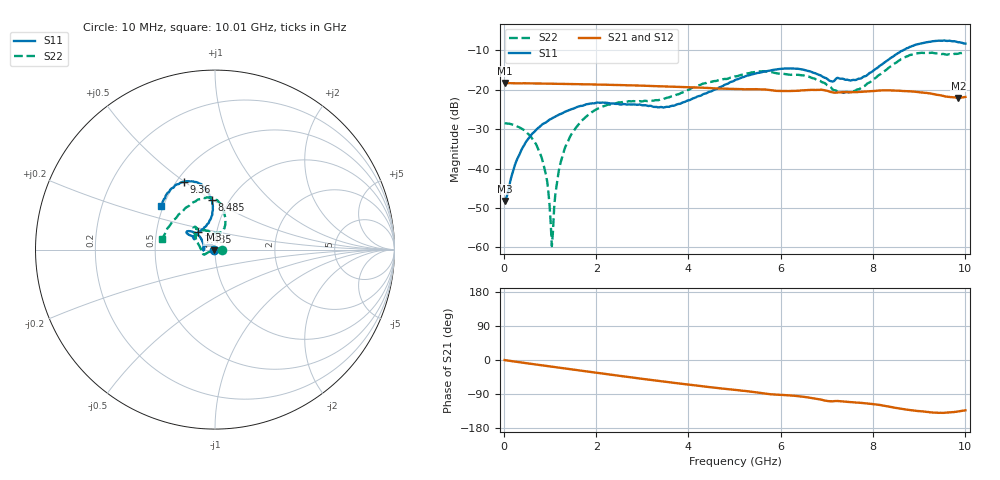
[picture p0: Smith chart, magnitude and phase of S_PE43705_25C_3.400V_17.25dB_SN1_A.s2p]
! Device ID: PE43705
! Serial: 1
! Insertion: A
! Impedance: 50 ohm
! Temp: 25C
! VDD: 3.400V
! Attenuation Step: 17.25dB
#  Hz  S  RI  R  50
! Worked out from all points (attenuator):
!   401 points, 10 MHz to 10.01 GHz, reference 50 ohm
!   highest |S21| = -18.31 dB at 10 MHz (marker M1); lowest = -22.1 dB at 9.86 GHz (marker M2)
!   lowest |S11| = -48.2 dB at 10 MHz (marker M3), VSWR 1.01, Z = 49.6 + j0.0457 ohm
!   |S11| at or under -10 dB: start of sweep to 8.659 GHz
!   |S22| runs from -59.7 to -10.4 dB; largest |S21 - S12| = 0.0015
!   S11 on the Smith chart (normalised r, x): 10 MHz: 0.99, +0.00; 7.435 GHz: 0.82, +0.16; 8.485 GHz: 0.83, +0.49; 9.36 GHz: 0.55, +0.50; 10.01 GHz: 0.49, +0.27
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1e7  -0.00385 0.000461  0.1214 -0.000448  0.1216 -0.000501  0.0375 1.82e-05
3.35e8  -0.00617 0.0139  0.1199 -0.0124  0.1197 -0.0123  0.033 0.00418
7.1e8  -0.0187 0.0255  0.1173 -0.0254  0.1173 -0.0253  0.0184 0.00605
8.85e8  -0.0268 0.0268  0.1155 -0.0314  0.1155 -0.0313  0.00893 0.0036
1.01e9  -0.0324 0.0273  0.1138 -0.0356  0.1139 -0.0355  0.00158 0.00133
1.035e9  -0.0334 0.0272  0.1134 -0.0363  0.1135 -0.0363  0.000146 0.00103
1.085e9  -0.0358 0.0269  0.1128 -0.0377  0.1128 -0.0378  -0.00315 -0.000261
1.16e9  -0.039 0.0266  0.1119 -0.0401  0.1118 -0.0401  -0.00732 -0.00166
1.26e9  -0.0432 0.0254  0.1104 -0.0433  0.1105 -0.0432  -0.0133 -0.00406
1.435e9  -0.0513 0.0227  0.1076 -0.0487  0.1077 -0.0486  -0.0242 -0.00858
1.685e9  -0.0601 0.0168  0.1032 -0.0558  0.1033 -0.0559  -0.0376 -0.0153
2.26e9  -0.0676 0.000283  0.0912 -0.0709  0.0912 -0.0707  -0.0584 -0.0277
3.36e9  -0.0596 0.0035  0.063 -0.0911  0.0628 -0.0909  -0.0739 -0.00399
5.01e9  -0.1001 0.0865  0.0196 -0.1002  0.0197 -0.1001  -0.1136 0.0937
6.01e9  -0.1535 0.1016  -0.00328 -0.0962  -0.00292 -0.0961  -0.104 0.1206
6.685e9  -0.1445 0.0819  -0.0182 -0.0978  -0.0184 -0.0977  -0.0853 0.112
7.435e9  -0.0919 0.0975  -0.0324 -0.0874  -0.0322 -0.0874  0.00894 0.0935
8.36e9  -0.0121 0.2454  -0.0537 -0.0823  -0.0536 -0.0825  0.0556 0.1845
8.485e9  -0.0183 0.2754  -0.0574 -0.0788  -0.0571 -0.0795  0.0496 0.2118
9.36e9  -0.1713 0.3772  -0.0658 -0.057  -0.0657 -0.0574  -0.1126 0.2668
9.86e9  -0.2772 0.2873  -0.0565 -0.0549  -0.0569 -0.055  -0.256 0.1282
1.001e10  -0.3008 0.2402  -0.055 -0.0595  -0.0557 -0.0588  -0.2947 0.0618
